(* Logix 5000 AddOnInstructionDefinition export AMCI_5034_PTO_AM_MAJ; software revision 37.00 *)

TYPE AMCI_5034_PTO_AM_Input_Data :
STRUCT
   ConnectionFaulted : DINT;
   MovingCW : BOOL;
   MovingCCW : BOOL;
   InHoldState : BOOL;
   Stopped : BOOL;
   AtHome : BOOL;
   Accelerating : BOOL;
   Decelerating : BOOL;
   MoveComplete : BOOL;
   HomeInvalid : BOOL;
   InvalidProfile : BOOL;
   PositionInvalid : BOOL;
   InputError : BOOL;
   CommandError : BOOL;
   ConfigurationError : BOOL;
   ModuleOK : BOOL;
   GeneralPurposeOutputStatus : BOOL;
   Input1Active : BOOL;
   Input2Active : BOOL;
   Input3Active : BOOL;
   Input4Active : BOOL;
   bit_20_reserved : BOOL;
   bit_21_reserved : BOOL;
   bit_22_reserved : BOOL;
   EncoderFollowerMode : BOOL;
   BlendMoveRunning : BOOL;
   BlendMoveAcknowledge : BOOL;
   MinimumRegistrationProgrammed : BOOL;
   EncoderMotionDirection : BOOL;
   MultipleInputsWithSameFunction : BOOL;
   FSCExceedsNumberOfDataBits : BOOL;
   AbsoluteEncoderSetupError : BOOL;
   bit_31_reserved : BOOL;
   CurrentPosition : DINT;
   EncoderPosition : DINT;
   CapturedPosition : DINT;
END_STRUCT
END_TYPE

TYPE AMCI_5034_PTO_AM_Output_Data :
STRUCT
   Command_Word : DINT;
   TargetPosition : DINT;
   TargetVelocity : UDINT;
   Acceleration : DINT;
   Deceleration : DINT;
END_STRUCT
END_TYPE

ADD_ON_INSTRUCTION AMCI_5034_PTO_AM_MAJ   (* revision 1.0, vendor AMCI, ExecuteEnableInFalse *)
// AMCI Jog
// Revision note:
// 10/01/2025  Initial release of AOI.  Making the rung false will NOT STOP THE JOG.
// Help:
// Performs Positive CW or Negative CCW Jog Moves
// AXIS INPUT DATA:  Input data from the AMCI 5034-PTO-AM.   Uses the AMCI_5034_PTO_Input_Data User Defined Data Type.
// AXIS OUTPUT DATA; Output data from the AOI to the AMCI 5034-PTO-AM.    Uses the AMCI_5034_PTO_Output_Data User Defined Data Type.
// DIRECTION: 0 for Positive CW Jog or 1 for Negative CCW Jog
// TARGETVELOCITY: Speed of move in units of steps / sec
// ACCELERATION: Acceleration Rate in units of steps / sec / ms
// DECELERATION:  Deceleration Rate in units of steps / sec / ms
// EN (Enable) Set when rung is true, Reset when rung is false
// DN (Done) Set when command is sent to the motion device.  Reset when the rung is false.
// ER (Error) Set when a command or input error failed to clear.  Reset when the rung is false.
// IP (In Process) Set when motion is occurring.   Reset when motion stops or the rung goes false.
VAR_IN_OUT
   Axis_Input_Data : AMCI_5034_PTO_AM_Input_Data; {required}
   Axis_Output_Data : AMCI_5034_PTO_AM_Output_Data; {required}
END_VAR
VAR_INPUT
   Direction_0_PositiveCW_1_NegativeCCW : BOOL; {required}   // 0=jog CW 1=jog CCW
   _0_normal_1_S_Curve_Acceleration : BOOL;
   _0_Triangular_1_Trapezoidal_S_Curve : BOOL;
   TargetVelocity : DINT; {required}
   Acceleration : DINT; {required}
   Deceleration : INT; {required}
END_VAR
VAR_OUTPUT
   EN : BOOL; {visible}   // set when rung with AOI is true
   DN : BOOL; {access Read Only, visible}   // set when move was succesfully initiated
   ER : BOOL; {visible}
   IP : BOOL; {visible}   // set when motion occurring
END_VAR
VAR
   command_data_block : DINT[5];
        [0]   // Command Word
        [1]   // Target Positon
        [2]   // Programmed Speed
        [3]   // Acceleration
        [4]   // Deceleration
   motion_occurring : BOOL; {access None}
   Internal_Enable : BOOL; {access None}   // set when driver ready to receive motion command
END_VAR

ROUTINE EnableInFalse   (* ladder *)
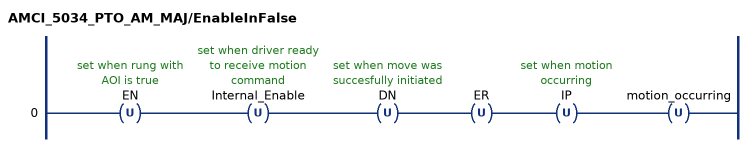
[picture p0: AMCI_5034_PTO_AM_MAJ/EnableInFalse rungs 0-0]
   0: OTU(EN)OTU(Internal_Enable)OTU(DN)OTU(ER)OTU(IP)OTU(motion_occurring);
END_ROUTINE

ROUTINE Logic   (* ladder *)
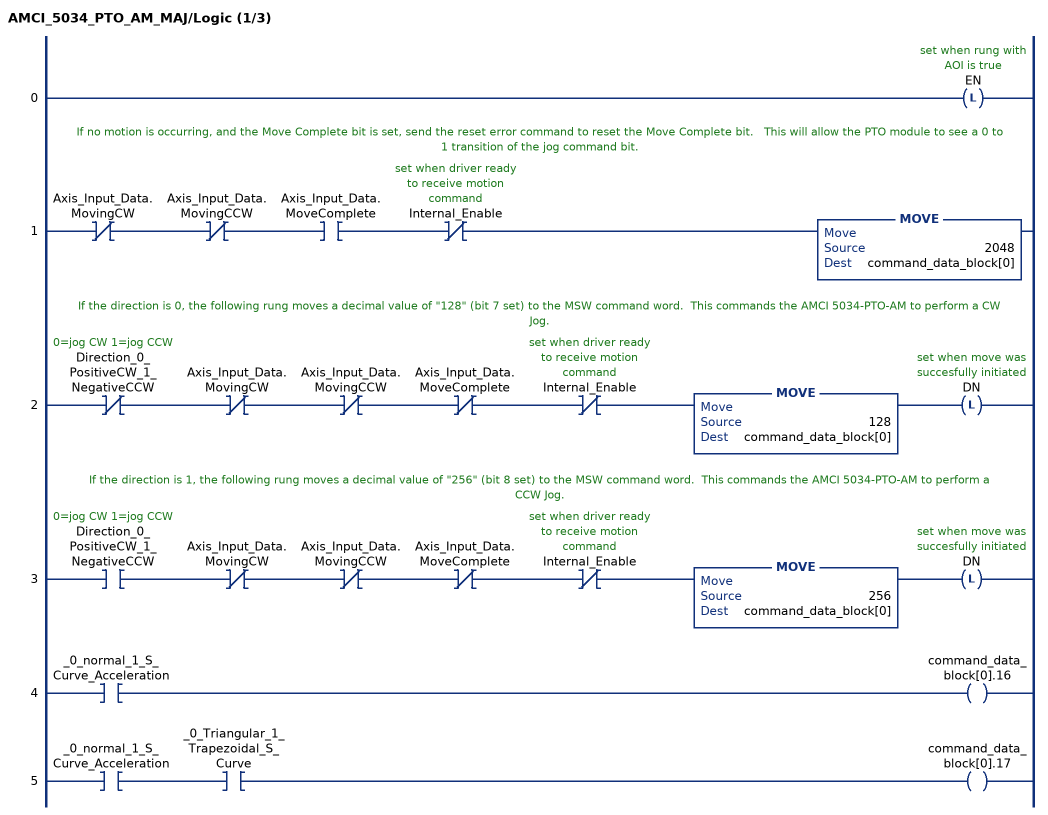
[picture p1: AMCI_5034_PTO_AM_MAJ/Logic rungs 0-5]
   0: OTL(EN);
   // If no motion is occurring, and the Move Complete bit is set, send the reset error command to reset the Move Complete bit.   This will allow the PTO module to see a 0 to 1 transition of the jog command bit.
   1: XIO(Axis_Input_Data.MovingCW)XIO(Axis_Input_Data.MovingCCW)XIC(Axis_Input_Data.MoveComplete)XIO(Internal_Enable)MOVE(2048,command_data_block[0]);
   // If the direction is 0, the following rung moves a decimal value of "128" (bit 7 set) to the MSW command word.  This commands the AMCI 5034-PTO-AM to perform a CW Jog.
   2: XIO(Direction_0_PositiveCW_1_NegativeCCW)XIO(Axis_Input_Data.MovingCW)XIO(Axis_Input_Data.MovingCCW)XIO(Axis_Input_Data.MoveComplete)XIO(Internal_Enable)MOVE(128,command_data_block[0])OTL(DN);
   // If the direction is 1, the following rung moves a decimal value of "256" (bit 8 set) to the MSW command word.  This commands the AMCI 5034-PTO-AM to perform a CCW Jog.
   3: XIC(Direction_0_PositiveCW_1_NegativeCCW)XIO(Axis_Input_Data.MovingCW)XIO(Axis_Input_Data.MovingCCW)XIO(Axis_Input_Data.MoveComplete)XIO(Internal_Enable)MOVE(256,command_data_block[0])OTL(DN);
   4: XIC(_0_normal_1_S_Curve_Acceleration)OTE(command_data_block[0].16);
   5: XIC(_0_normal_1_S_Curve_Acceleration)XIC(_0_Triangular_1_Trapezoidal_S_Curve)OTE(command_data_block[0].17);
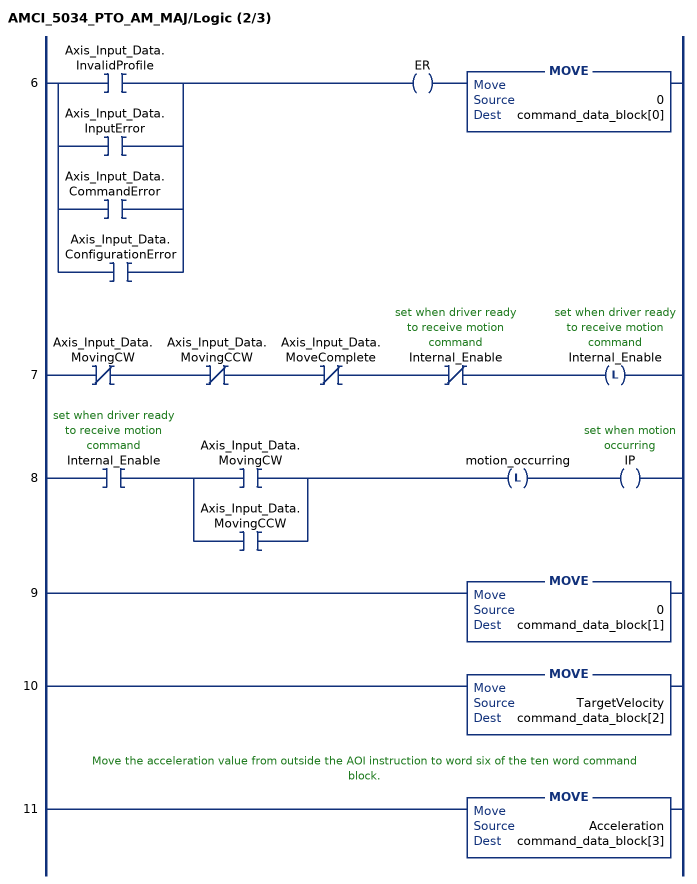
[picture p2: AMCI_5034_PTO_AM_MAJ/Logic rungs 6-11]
   6: [XIC(Axis_Input_Data.InvalidProfile) ,XIC(Axis_Input_Data.InputError) ,XIC(Axis_Input_Data.CommandError) ,XIC(Axis_Input_Data.ConfigurationError) ]OTE(ER)MOVE(0,command_data_block[0]);
   7: XIO(Axis_Input_Data.MovingCW)XIO(Axis_Input_Data.MovingCCW)XIO(Axis_Input_Data.MoveComplete)XIO(Internal_Enable)OTL(Internal_Enable);
   8: XIC(Internal_Enable)[XIC(Axis_Input_Data.MovingCW) ,XIC(Axis_Input_Data.MovingCCW) ]OTL(motion_occurring)OTE(IP);
   9: MOVE(0,command_data_block[1]);
   10: MOVE(TargetVelocity,command_data_block[2]);
   // Move the acceleration value from outside the AOI instruction to word six of the ten word command block.
   11: MOVE(Acceleration,command_data_block[3]);
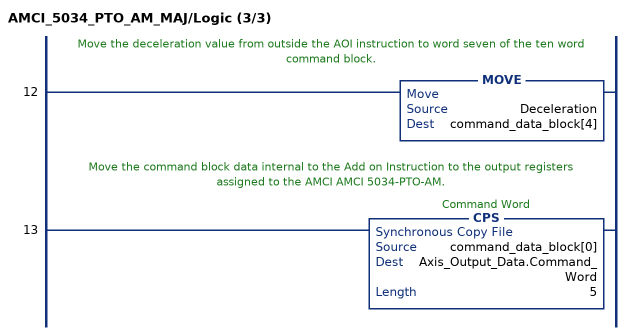
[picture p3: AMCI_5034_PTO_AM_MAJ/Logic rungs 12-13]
   // Move the deceleration value from outside the AOI instruction to word seven of the ten word command block.
   12: MOVE(Deceleration,command_data_block[4]);
   // Move the command block data internal to the Add on Instruction to the output registers assigned to the AMCI AMCI 5034-PTO-AM.
   13: CPS(command_data_block[0],Axis_Output_Data.Command_Word,5);
END_ROUTINE
END_ADD_ON_INSTRUCTION
